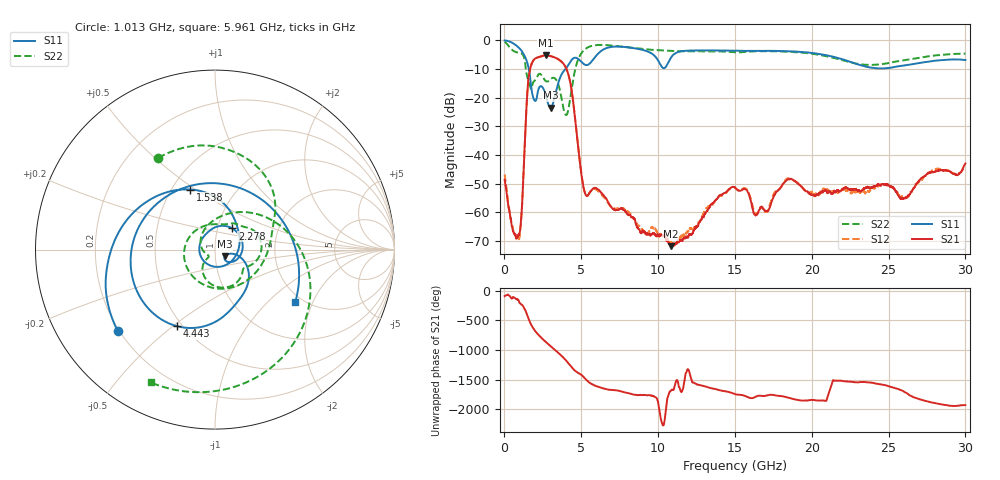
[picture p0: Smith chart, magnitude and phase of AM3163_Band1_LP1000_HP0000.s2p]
!Agilent Technologies,E8364B,MY43040894,A.07.50.67
!Agilent E8364B: A.07.50.67
!Date: Thursday, August 20, 2020 11:30:56
!Correction: S11(Full 2 Port(1,2))
!S21(Full 2 Port(1,2))
!S12(Full 2 Port(1,2))
!S22(Full 2 Port(1,2))
!S2P File: Measurements: S11, S21, S12, S22:
# Hz S  dB  R 50
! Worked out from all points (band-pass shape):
!   3201 points, 10 MHz to 30 GHz, reference 50 ohm
!   highest |S21| = -5.31 dB at 2.69 GHz (marker M1); lowest = -71.8 dB at 10.83 GHz (marker M2)
!   |S21| within 3 dB of the highest: 1.761 GHz to 3.857 GHz (2.095 GHz wide, 74.6 % of centre)
!   lowest |S11| = -23.5 dB at 3 GHz (marker M3), VSWR 1.14, Z = 55.7 - j4.18 ohm
!   |S11| at or under -10 dB: 1.587 GHz to 3.977 GHz (2.39 GHz wide, 85.9 % of centre)
!   |S22| runs from -26.1 to -0.6 dB; largest |S21 - S12| = 0.0089
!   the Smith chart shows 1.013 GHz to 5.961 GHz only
!   S11 on the Smith chart (normalised r, x): 1.013 GHz: 0.19, -0.35; 1.538 GHz: 0.62, +0.48; 2.278 GHz: 1.18, +0.28; 4.443 GHz: 0.47, -0.52; 5.961 GHz: 1.82, -1.50
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1e7  -0.07 -8.6  -48.60 -86.8  -46.82 -159.8  -0.56 -22.6
5.441969e8  -1.00 -72.5  -66.36 -105.7  -65.42 122.8  -3.55 -148.1
1.012791e9  -3.01 -140.1  -66.52 151.8  -66.97 -0.0  -4.43 121.7
1.537616e9  -8.84 112.2  -14.91 -90.1  -14.89 -90.1  -13.78 -109.8
1.912491e9  -20.58 -100.4  -6.80 74.1  -6.80 74.1  -14.39 46.9
2.277994e9  -16.34 50.5  -5.78 -40.9  -5.78 -41.0  -11.69 8.5
2.690356e9  -19.26 -40.1  -5.31 -143.2  -5.32 -143.2  -14.24 -31.2
2.999628e9  -23.50 -34.0  -5.53 146.7  -5.54 146.6  -13.60 -46.0
3.590056e9  -13.49 -30.1  -6.93 13.5  -6.95 13.6  -16.98 -118.8
4.442897e9  -6.45 -116.1  -20.18 129.2  -20.14 129.3  -14.73 82.4
5.014581e9  -7.55 146.7  -47.05 19.0  -46.81 18.9  -4.46 -28.1
5.961141e9  -5.44 -33.3  -51.61 -168.3  -52.02 -169.3  -1.70 -115.8
6.635916e9  -2.75 -105.3  -55.30 138.0  -55.93 137.0  -1.70 -157.0
7.619962e9  -2.25 -172.7  -58.73 99.6  -58.59 98.5  -2.23 155.4
1.000979e10  -7.13 68.4  -68.25 -102.0  -68.01 -32.2  -3.50 61.3
1.082514e10  -6.15 81.5  -71.80 115.9  -70.53 111.9  -3.72 32.1
1.25402e10  -3.55 3.2  -65.13 -143.0  -64.78 -122.7  -3.87 -24.7
1.5005e10  -3.62 -72.0  -51.36 55.9  -51.34 57.6  -4.22 -93.2
2.000958e10  -4.41 163.3  -53.92 -41.5  -52.94 -57.8  -4.71 136.6
2.275554e10  -8.00 60.3  -52.01 -102.1  -52.68 -96.4  -7.98 21.3
2.500479e10  -9.67 -62.2  -50.52 -168.6  -50.85 -170.1  -7.96 -92.2
3e10  -6.90 104.9  -42.99 -130.9  -44.16 -130.1  -4.66 102.6
